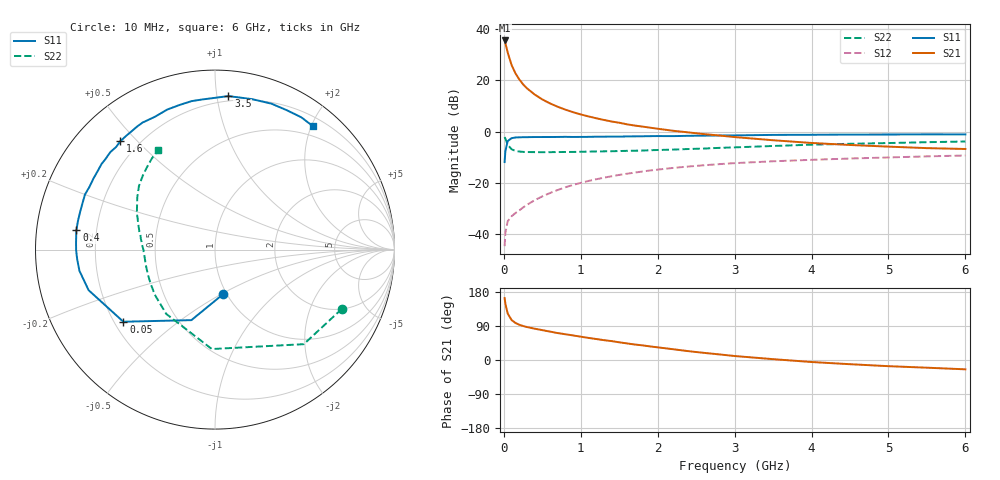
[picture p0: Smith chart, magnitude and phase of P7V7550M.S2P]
! SIEMENS Small Signal Semiconductors
! BFP196
! Si NPN RF Bipolar Junction Transistor in SOT143
! VCE = 0.75 V  IC = 50 mA
! Common Emitter S-Parameters:  May  1996
# GHz  S  MA  R  50
!  f  S11  S21  S12  S22
! GHz  MAG  ANG  MAG  ANG  MAG  ANG  MAG  ANG
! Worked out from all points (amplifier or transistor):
!   36 points, 10 MHz to 6 GHz, reference 50 ohm
!   highest |S21| = 35.6 dB at 10 MHz (marker M1)
!   |S21| within 3 dB of that: start of sweep to 35.96 MHz
!   unconditionally stable (mu >= 1): 347.4 MHz to end of sweep
!   at 250 MHz: K = 0.91, MSG = 24.1 dB, |S12| = -29.7 dB
!   at 1.4 GHz: K = 1.12, MAG = 8.6 dB, |S12| = -17.5 dB
!   at 6 GHz: K = 1.04, MAG = 0.1 dB, |S12| = -9.4 dB
!   S11 on the Smith chart (normalised r, x): 10 MHz: 0.96, -0.51; 50 MHz: 0.24, -0.33; 400 MHz: 0.12, +0.07; 1.6 GHz: 0.13, +0.45; 3.5 GHz: 0.17, +1.08; 6 GHz: 0.34, +2.02
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0.01  0.2524 -79.7  60.58 163.4  0.0057 72.7  0.7799 -25.1
0.02  0.4144 -108.5  53.6 148.4  0.0104 62.3  0.7227 -46.8
0.05  0.6498 -141.8  35.25 122.7  0.0175 46.0  0.5543 -91.8
0.1  0.7396 -162.2  20.14 105.6  0.0219 42.8  0.4495 -127.2
0.15  0.7645 -171.1  13.85 97.9  0.0253 45.1  0.4191 -143.2
0.2  0.7697 -176.0  10.5 93.0  0.0285 48.9  0.4055 -152.3
0.25  0.7736 -179.6  8.399 89.7  0.0326 51.9  0.3997 -158.4
0.3  0.7751 177.3  7.027 87.0  0.0367 54.8  0.3967 -162.2
0.4  0.78 172.1  5.304 82.7  0.0452 58.5  0.3948 -167.8
0.5  0.78 168.1  4.248 78.8  0.0537 60.3  0.3939 -171.5
0.6  0.7803 164.3  3.549 74.9  0.0626 61.0  0.3944 -174.1
0.7  0.7827 160.1  3.055 71.1  0.0716 61.2  0.396 -176.2
0.9  0.782 153.5  2.39 64.8  0.09 60.1  0.3985 -179.8
1.1  0.7862 146.6  1.976 58.3  0.1077 58.1  0.4046 177.5
1.3  0.7921 140.1  1.687 52.4  0.1249 55.6  0.4091 174.8
1.6  0.8019 131.1  1.384 43.8  0.1492 51.3  0.4186 171.3
2.2  0.8122 114.3  1.034 28.4  0.1937 42.0  0.4429 163.7
2.8  0.8374 99.0  0.836 14.8  0.2299 32.6  0.4785 155.4
3.5  0.8585 85.0  0.675 2.2  0.2614 22.3  0.5212 146.2
4.5  0.8717 68.9  0.545 -11.1  0.2961 10.1  0.5751 134.5
5.5  0.8801 56.9  0.473 -20.3  0.3261 -0.6  0.6178 124.7
6  0.8778 51.6  0.455 -24.6  0.3394 -6.3  0.6377 119.8
